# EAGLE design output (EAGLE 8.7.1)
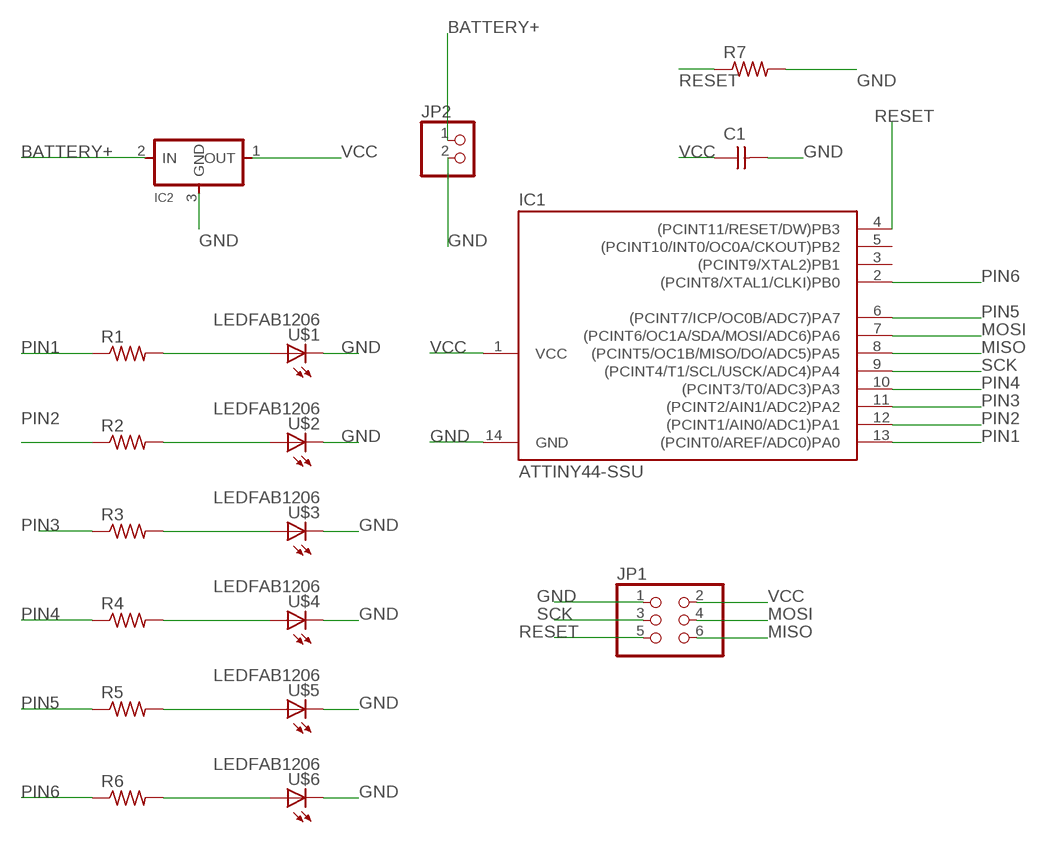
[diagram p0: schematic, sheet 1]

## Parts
C1  CAP-UNPOLARIZEDFAB  [C1206FAB]
IC1  ATTINY44-SSU  [SOIC14]
IC2  REGULATORSOT23  [SOT23]
JP1  PINHD-2X3-SMD  [2X03SMD]
JP2  PINHD-1X2  [1X02]
R1  RES-US1206FAB  [R1206FAB]
R2  RES-US1206FAB  [R1206FAB]
R3  RES-US1206FAB  [R1206FAB]
R4  RES-US1206FAB  [R1206FAB]
R5  RES-US1206FAB  [R1206FAB]
R6  RES-US1206FAB  [R1206FAB]
R7  RES-US1206W  [R1206W]
U$1  LEDFAB1206  [LED1206FAB]
U$2  LEDFAB1206  [LED1206FAB]
U$3  LEDFAB1206  [LED1206FAB]
U$4  LEDFAB1206  [LED1206FAB]
U$5  LEDFAB1206  [LED1206FAB]
U$6  LEDFAB1206  [LED1206FAB]

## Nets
BATTERY+: IC2.2(IN) JP2.1
GND: C1.2 IC1.14(GND) IC2.3(GND) JP1.1 JP2.2 R7.2 U$1.2(C) U$2.2(C) U$3.2(C) U$4.2(C) U$5.2(C) U$6.2(C)
MISO: IC1.8((PCINT5/OC1B/MISO/DO/ADC5)PA5) JP1.6
MOSI: IC1.7((PCINT6/OC1A/SDA/MOSI/ADC6)PA6) JP1.4
N$2: R1.2 U$1.1(A)
N$4: R2.2 U$2.1(A)
N$6: R3.2 U$3.1(A)
N$8: R4.2 U$4.1(A)
N$10: R5.2 U$5.1(A)
N$12: R6.2 U$6.1(A)
PIN1: IC1.13((PCINT0/AREF/ADC0)PA0) R1.1
PIN2: IC1.12((PCINT1/AIN0/ADC1)PA1) R2.1
PIN3: IC1.11((PCINT2/AIN1/ADC2)PA2) R3.1
PIN4: IC1.10((PCINT3/T0/ADC3)PA3) R4.1
PIN5: IC1.6((PCINT7/ICP/OC0B/ADC7)PA7) R5.1
PIN6: IC1.2((PCINT8/XTAL1/CLKI)PB0) R6.1
RESET: IC1.4((PCINT11/RESET/DW)PB3) JP1.5 R7.1
SCK: IC1.9((PCINT4/T1/SCL/USCK/ADC4)PA4) JP1.3
VCC: C1.1 IC1.1(VCC) IC2.1(OUT) JP1.2
Unconnected: IC1.3((PCINT9/XTAL2)PB1) IC1.5((PCINT10/INT0/OC0A/CKOUT)PB2)

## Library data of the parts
C1 = fab:CAP-UNPOLARIZED
IC1 = fab:ATTINY44
IC2 = fab:REGULATOR
JP1 = fab:PINHD-2X3-SMD: PIN HEADER
JP2 = pinhead:PINHD-1X2: PIN HEADER
R1-R7 = fab:RES-US: Resistor (US Symbol)
U$1-U$6 = fab:LED: LED

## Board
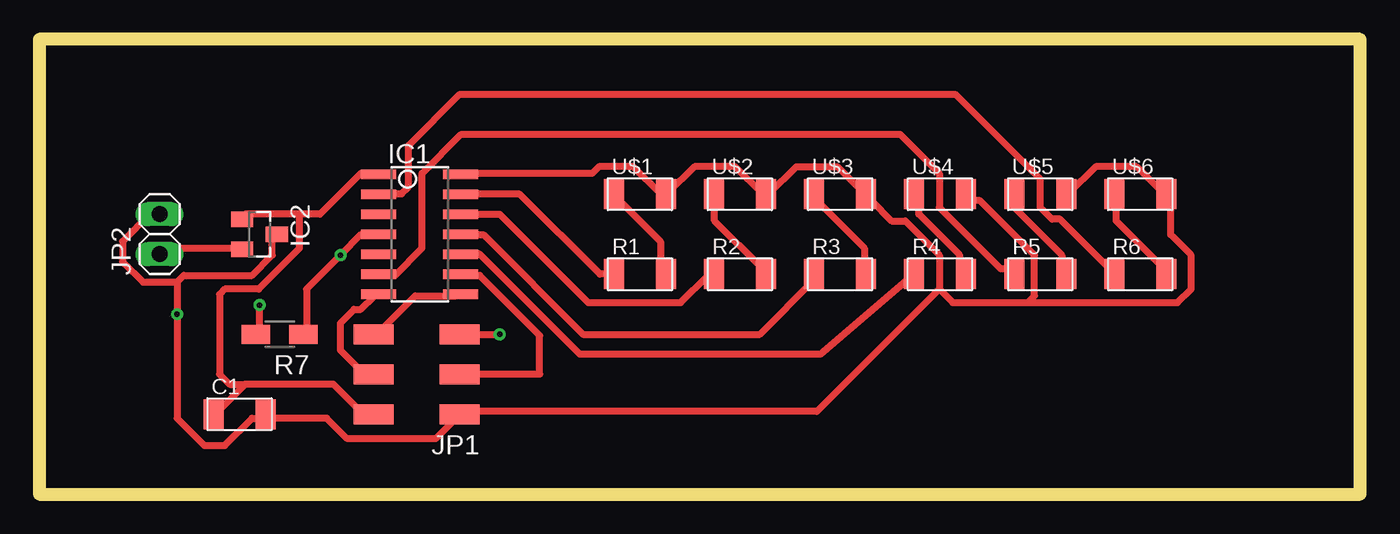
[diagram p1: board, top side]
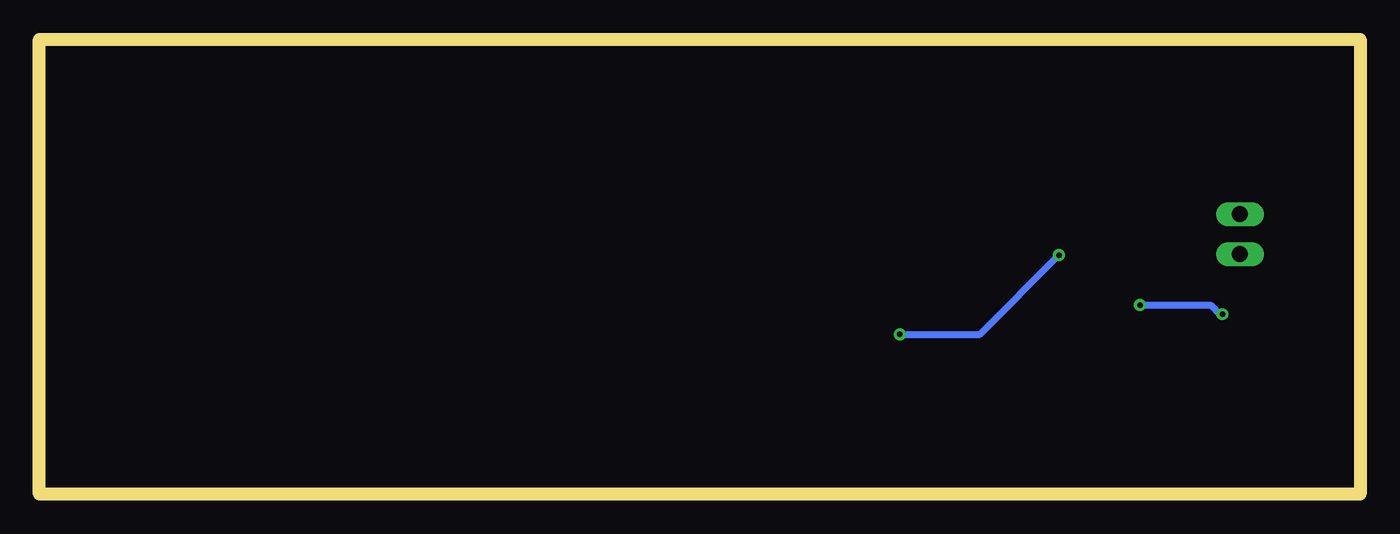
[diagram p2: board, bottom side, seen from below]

Size 83.8 x 28.88 mm. Coordinates in mm from the lower left corner, seen from the top.
Outline: 0,0 83.8,0 83.8,28.88 0,28.88 0,0
Copper layers (1*16): Top 0.035mm / dielectric 1.5mm / Bottom 0.035mm
Design rules "default *": minimum track width 18mil, minimum drill 0.35mm, track to track 16mil, track to pad 16mil, pad to pad 16mil, via to via 16mil, smd to smd 16mil, copper to edge 40mil, drill to drill 6mil, minimum pad ring 10mil, minimum via ring 8mil, stop-mask expansion 4mil, vias tented up to drill 0mil, thermal gap 10mil

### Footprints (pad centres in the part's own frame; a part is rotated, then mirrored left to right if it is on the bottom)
C1206FAB = smd 1.27 x 1.905: 1 -1.651,0; 2 1.651,0
SOIC14 = smd 0.61 x 2.21: 1 -3.81,-2.603; 2 -2.54,-2.603; 3 -1.27,-2.603; 4 0,-2.603; 5 1.27,-2.603; 6 2.54,-2.603; 7 3.81,-2.603; 8 3.81,2.603; 9 2.54,2.603; 10 1.27,2.603; 11 0,2.603; 12 -1.27,2.603; 13 -2.54,2.603; 14 -3.81,2.603
SOT23 = smd 1 x 1.4: 1 -0.95,-1.1; 2 0.95,-1.1; 3 0,1.1
2X03SMD = smd 2.54 x 1.27: 1 -2.54,2.54; 2 2.92,2.54; 3 -2.54,0; 4 2.92,0; 5 -2.54,-2.54; 6 2.92,-2.54
1X02 = drill 1.016 long: 1 -1.27,0; 2 1.27,0
R1206FAB = smd 1.27 x 1.905: 1 -1.651,0; 2 1.651,0
R1206W = smd 1.8 x 1.2: 1 -1.499,0; 2 1.499,0
LED1206FAB = smd 1.27 x 1.905: 1 -1.651,0; 2 1.651,0

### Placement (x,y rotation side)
C1  12.7,5.08 0 top
IC1  24.13,16.51 270 top
IC2  13.97,16.51 270 top
JP1  24.13,7.62 180 top
JP2  7.62,16.51 90 top
R1  38.1,13.97 0 top
R2  44.45,13.97 0 top
R3  50.8,13.97 0 top
R4  57.15,13.97 0 top
R5  63.5,13.97 0 top
R6  69.85,13.97 0 top
R7  15.24,10.16 180 top
U$1  38.1,19.05 0 top
U$2  44.45,19.05 0 top
U$3  50.8,19.05 0 top
U$4  57.15,19.05 0 top
U$5  63.5,19.05 0 top
U$6  69.85,19.05 0 top

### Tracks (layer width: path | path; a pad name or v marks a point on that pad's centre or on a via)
BATTERY+
  Top 0.457: IC2.2 12.62,15.62 7.87,15.62 JP2.1
GND  (via drill 0.35)
  Top 0.457: 14.35,4.83 18.24,4.83 19.53,3.53 25.15,3.53 26.44,4.83 JP1.1 26.87,5.26 49.33,5.26 57.1,13.03 | 8.74,13.46 9.17,13.89 13.49,13.89 14.78,15.19 14.78,16.48 IC2.3 | 8.74,13.46 6.58,13.46 5.28,14.76 5.28,16.05 7.01,17.78 JP2.2 | 14.35,4.83 13.49,4.83 11.76,3.1 10.46,3.1 8.74,4.83 v8.74,11.43 8.74,13.46 | 14.35,4.83 C1.2 | U$5.2 65.3,19.08 67.03,20.8 69.62,20.8 71.35,19.08 U$6.2 71.78,18.64 71.78,16.48 73.08,15.19 73.08,13.03 72.21,12.17 62.71,12.17 | 62.71,12.17 63.14,12.6 63.14,15.19 59.69,18.64 58.83,18.64 U$4.2 | 62.71,12.17 57.96,12.17 57.1,13.03 | 57.1,13.03 57.1,15.19 54.94,17.35 54.08,17.35 52.78,18.64 U$3.2 52.35,19.08 50.62,20.8 48.03,20.8 46.3,19.08 U$2.2 45.87,19.08 44.14,20.8 41.55,20.8 39.83,19.08 U$1.2 39.39,19.08 37.67,20.8 35.51,20.8 35.08,20.37 26.87,20.37 IC1.14 | R7.2 13.97,10.39 v13.97,12.02
  Bottom 0.457: v13.97,12.02 9.48,12.02 8.89,11.43 v8.74,11.43
MISO
  Top 0.457: IC1.8 26.44,12.6 23.85,12.6 21.26,10.01 JP1.6
MOSI
  Top 0.457: IC1.7 21.26,12.6 20.4,11.73 19.96,11.73 19.1,10.87 19.1,9.14 20.83,7.42 JP1.4
N$2
  Top 0.457: R1.2 39.39,14.33 39.39,16.05 36.8,18.64 U$1.1
N$4
  Top 0.457: U$2.1 42.85,18.64 42.85,17.35 45.87,14.33 R2.2
N$6
  Top 0.457: R3.2 52.35,14.33 52.35,15.62 49.33,18.64 U$3.1
N$8
  Top 0.457: U$4.1 55.8,18.64 55.8,17.78 58.39,15.19 58.39,14.33 R4.2
N$10
  Top 0.457: U$5.1 61.85,18.21 64.87,15.19 64.87,14.33 R5.2
N$12
  Top 0.457: U$6.1 68.33,18.64 68.33,17.35 71.35,14.33 R6.2
PIN1
  Top 0.457: R1.1 35.56,13.97 30.48,19.05 IC1.13
PIN2
  Top 0.457: IC1.12 29.21,17.78 34.82,12.17 40.69,12.17 42.42,13.89 R2.1
PIN3
  Top 0.457: 48.89,13.89 R3.1 49.15,13.59 45.72,10.16 34.49,10.16 28.17,16.48 26.87,16.48 IC1.11
PIN4
  Top 0.457: IC1.10 27.94,15.24 34.29,8.89 49.53,8.89 R4.1
PIN5
  Top 0.457: R5.1 61.85,14.33 60.98,14.33 57.1,18.21 57.1,20.37 54.61,22.86 26.77,22.86 24.28,20.37 24.28,15.62 22.55,13.89 21.69,13.89 IC1.6
PIN6
  Top 0.457: R6.1 67.89,14.33 64.76,17.46 64.25,17.46 63.5,18.22 63.5,20.02 58.11,25.4 26.67,25.4 23.42,22.15 23.42,19.51 22.99,19.08 21.69,19.08 IC1.2
RESET  (via drill 0.35)
  Top 0.457: R7.1 16.94,10.44 16.94,13.03 v19.1,15.19 20.4,16.48 21.26,16.48 IC1.4 | JP1.5 v29.21,10.16
  Bottom 0.457: v29.21,10.16 24.13,10.16 v19.1,15.19
SCK
  Top 0.457: IC1.9 26.87,13.89 27.94,13.89 31.75,10.08 31.75,7.62 27.08,7.62 26.87,7.42 JP1.3
VCC
  Top 0.457: 16.51,17.78 17.8,17.78 20.4,20.37 21.26,20.37 IC1.1 | 16.51,17.78 13.06,17.78 IC2.1 | 13.06,6.98 11.33,5.26 C1.1 | 13.06,6.98 18.67,6.98 20.83,4.83 JP1.2 | 16.51,17.78 16.51,15.62 13.92,13.03 11.76,13.03 11.43,12.7 11.43,7.62 12.06,6.98 13.06,6.98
